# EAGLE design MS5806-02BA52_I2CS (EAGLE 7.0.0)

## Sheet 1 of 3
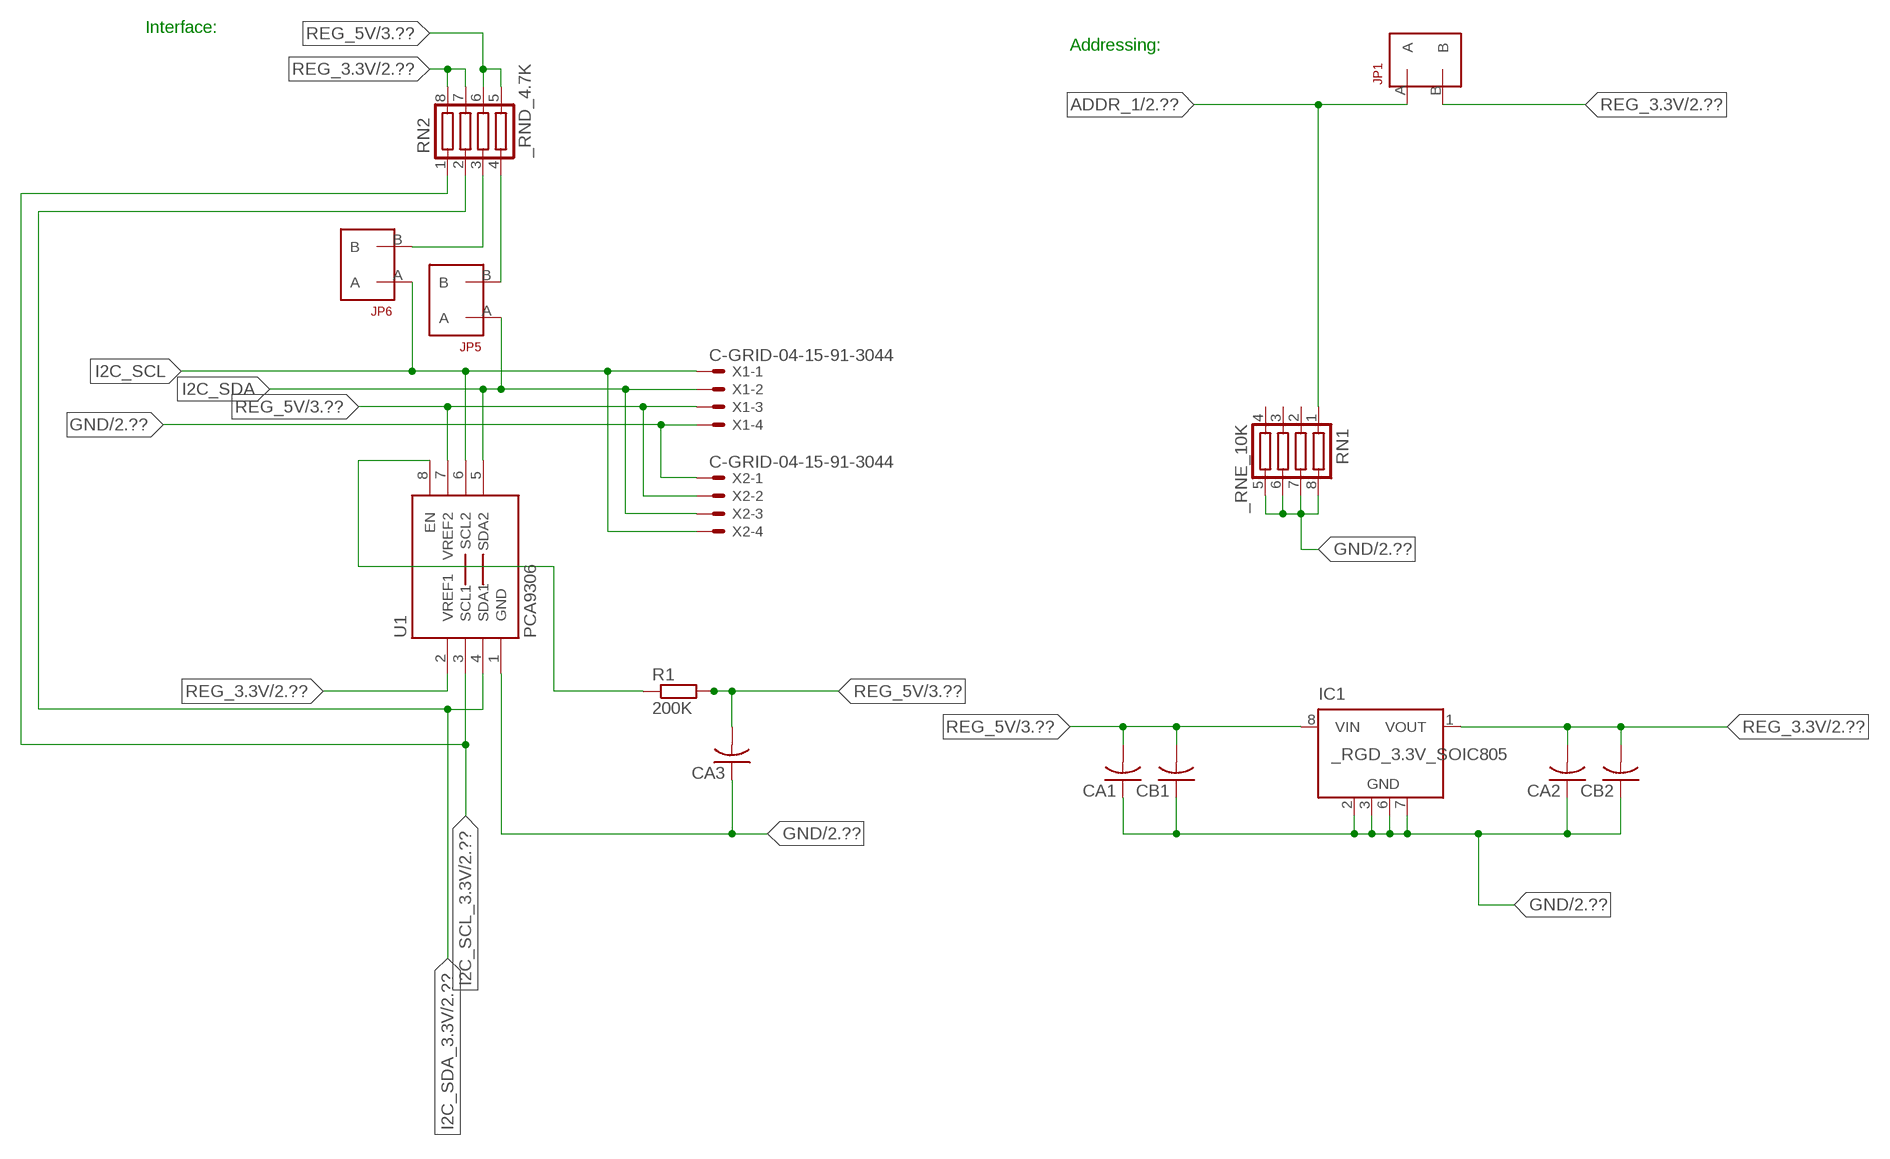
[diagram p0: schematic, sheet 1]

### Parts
CA1  CC1206KRX7R9BB104  [.1UF]
CA2  CC1206KRX7R9BB104  [.1UF]
CA3  CC1206KRX7R9BB104  [.1UF]
CB1  TMK316F106ZL-TC1206K  [TMK316F106ZL-T]
CB2  TMK316F106ZL-TC1206K  [TMK316F106ZL-T]
IC1  _RGD_3.3V_SOIC805  [_RGC_3.3V_SOIC8]
JP1  JUMPER_1X2_2MM  [JUMPER_1X2_2MM]
JP5  JUMPER_1X2_2MM  [JUMPER_1X2_2MM]
JP6  JUMPER_1X2_2MM  [JUMPER_1X2_2MM]
R1  200K  RESISTOR_SMT-0603  [R603]
RN1  _RNE_10K  [RNE]
RN2  _RND_4.7K  [RND]
U1  PCA9306  PCA9306_NCD  [PSOP-8]
X1  C-GRID-04-15-91-3044  [15-91-04]
X2  C-GRID-04-15-91-3044  [15-91-04]

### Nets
ADDR_1: JP1.A RN1.1 ; also sheet 2
GND: CA1.1 CA2.1 CA3.1 CB1.1 CB2.1 IC1.2(GND) IC1.3(GND) IC1.6(GND) IC1.7(GND) RN1.5 RN1.6 RN1.7 RN1.8 U1.1(GND) X1.4 X2.1 ; also sheet 2,3
I2C_SCL: JP6.A U1.6(SCL2) X1.1 X2.4
I2C_SCL_3.3V: RN2.1 U1.3(SCL1) ; also sheet 2
I2C_SDA: JP5.A U1.5(SDA2) X1.2 X2.3
I2C_SDA_3.3V: RN2.2 U1.4(SDA1) ; also sheet 2
N$1: JP6.B RN2.3
N$2: JP5.B RN2.4
N$3: R1.1 U1.8(EN)
REG_3.3V: CA2.2 CB2.2 IC1.1(VOUT) JP1.B RN2.7 RN2.8 U1.2(VREF1) ; also sheet 2
REG_5V: CA1.2 CA3.2 CB1.2 IC1.8(VIN) R1.2 RN2.5 RN2.6 U1.7(VREF2) X1.3 X2.2 ; also sheet 3
Unconnected: IC1.4(NC) IC1.5(NC) RN1.2 RN1.3 RN1.4

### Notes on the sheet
- Interface:
- Addressing:

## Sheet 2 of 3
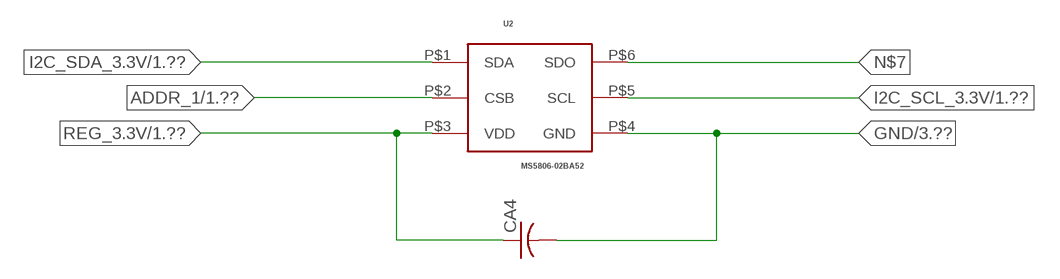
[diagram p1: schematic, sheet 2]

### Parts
CA4  _CA_.10UF_50VC1206K  [_CA_.1UF_50V]
U2  MS5806-02BA52  [MS5806-02BA52]

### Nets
ADDR_1: U2.P$2(CSB) ; also sheet 1
GND: CA4.2 U2.P$4(GND) ; also sheet 1,3
I2C_SCL_3.3V: U2.P$5(SCL) ; also sheet 1
I2C_SDA_3.3V: U2.P$1(SDA) ; also sheet 1
N$7: U2.P$6(SDO)
REG_3.3V: CA4.1 U2.P$3(VDD) ; also sheet 1

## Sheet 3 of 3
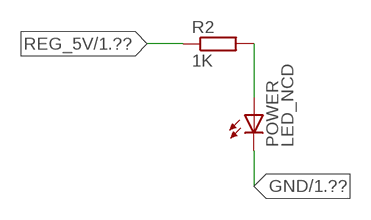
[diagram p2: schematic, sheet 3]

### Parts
POWER  LED_NCD  [CHIPLED_0603]
R2  1K  RESISTOR_SMT-0402  [R402]

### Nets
GND: POWER.C ; also sheet 1,2
N$4: POWER.A R2.2
REG_5V: R2.1 ; also sheet 1

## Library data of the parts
CA1-CA3 = NCD_ULTIMATE_LIBRARY:CC1206KRX7R9BB104: Capacitor CA .1uF 50V SMT C1206K CC1206KRX7R9BB104
CA4 = NCD_ULTIMATE_LIBRARY:_CA_.10UF_50V: Capacitor .1uF SMT
CB1 CB2 = NCD_ULTIMATE_LIBRARY:TMK316F106ZL-T: Capacitor CB 10uF SMT 1206 TMK316F106ZL-T
IC1 = NCD_ULTIMATE_LIBRARY:_RGD_3.3V_SOIC8: Regulator Linear 3.3V Chip Positive VOLTAGE REGULATOR Digikey 497-1199-2-ND/L78L33ACD13TR
JP1 JP5 JP6 = NCD_ULTIMATE_CONNECTORS:JUMPER_1X2_2MM
POWER = NCD_ULTIMATE_LIBRARY:LED_NCD: LED Digikey 754-1132-2-ND/APT2012SRCPRV
R1 R2 = NCD_ULTIMATE_LIBRARY:RESISTOR_SMT: NCD Resistor
RN1 = NCD_ULTIMATE_LIBRARY:_RNE_10K: Resistor Array RNE SMT 10K x 4 Single Resistor Source: http://www.ctscorp.com/components/Datasheets/CTSChipArrayDs.pdf Digikey 742C083103JPTR-ND/742C083103JP; OC_FARNELL: unknown; OC_NEWARK: unknown
RN2 = NCD_ULTIMATE_LIBRARY:_RND_4.7K: Resistor Array RND SMT 4.7K x 4 Single Resistor Source: http://www.ctscorp.com/components/Datasheets/CTSChipArrayDs.pdf Digikey 742C083472JPTR-ND/742C083472JP; OC_FARNELL: unknown; OC_NEWARK: unknown
U1 = NCD_ULTIMATE_LIBRARY:PCA9306_NCD: NCD Bidirectional I2C level shifter. NOT compatible with all available part number pinout schemes- DOUBLE CHECK!!!; PROD_ID: IC-10023
U2 = NCD_ULTIMATE_bhaskar:MS5806-02BA52
X1 X2 = NCD_ULTIMATE_CONNECTORS:C-GRID-04: CONNECTOR 4-Pos I2C wire to board 2.54 mm (0.100") pitch header Digikey WM1342-ND/0015912045; OC_FARNELL: unknown; OC_NEWARK: unknown

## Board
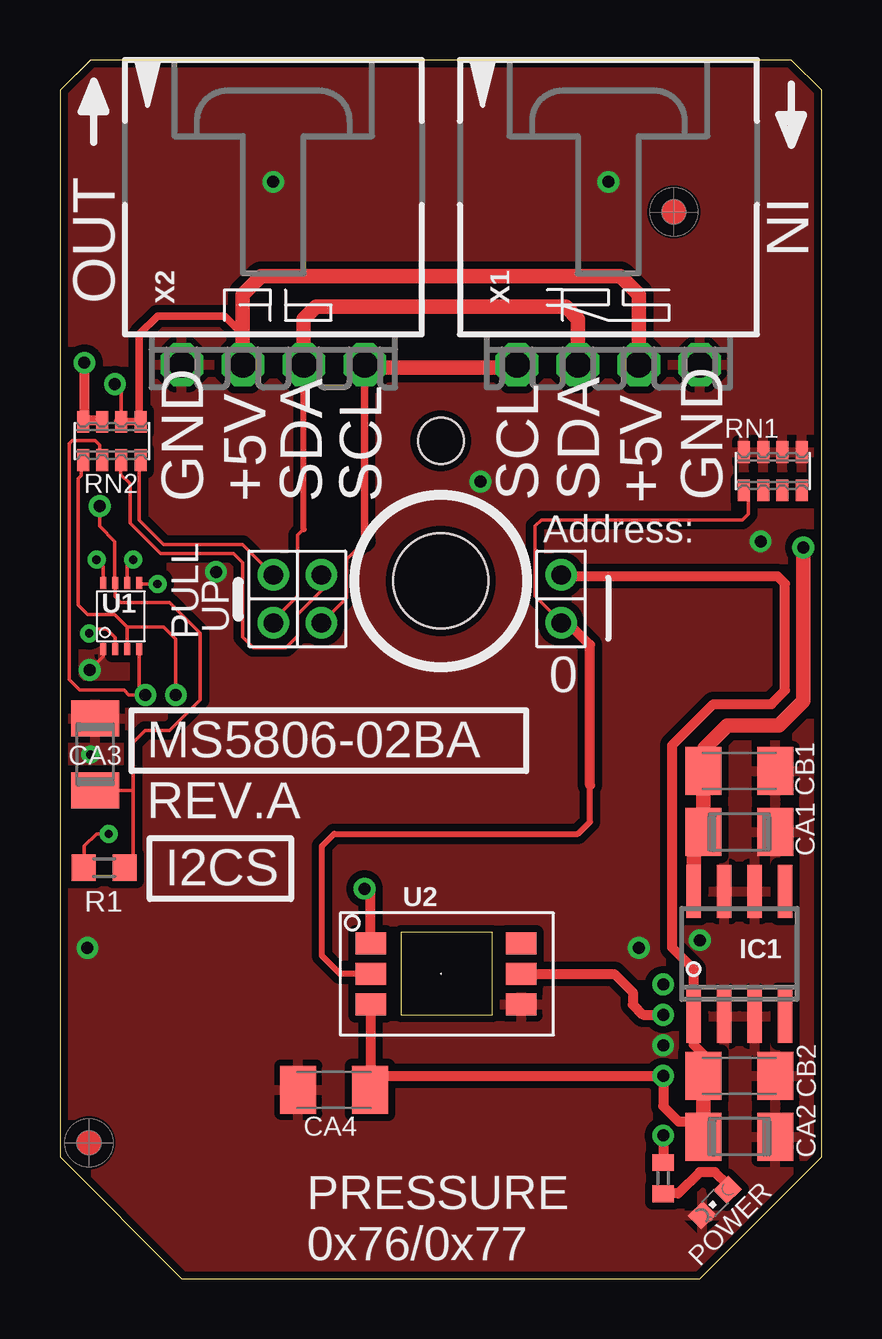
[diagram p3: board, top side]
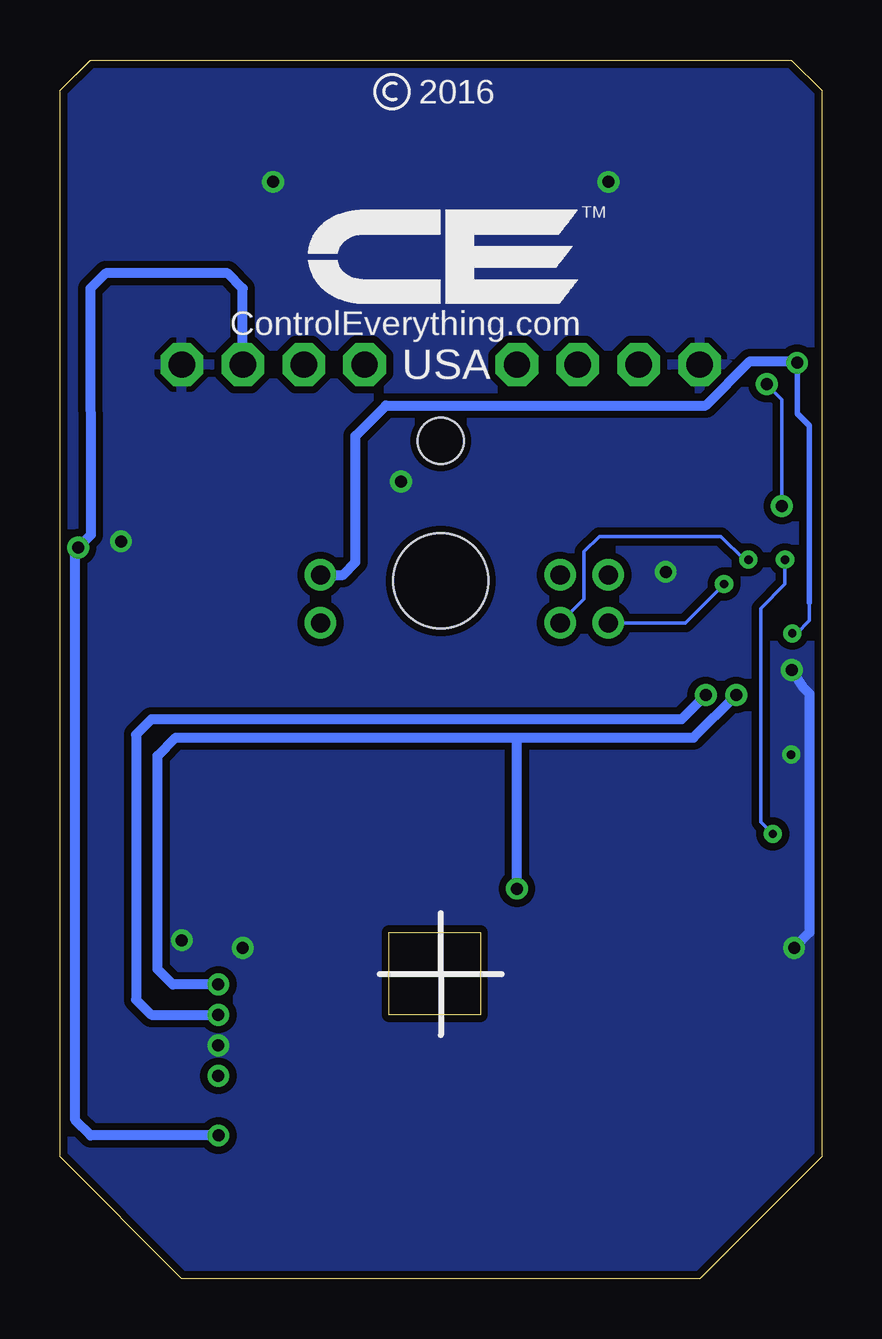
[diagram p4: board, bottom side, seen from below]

Size 31.75 x 50.8 mm. Coordinates in mm from the lower left corner, seen from the top.
Outline: 32 segments
Copper layers (1*16): Top 0.035mm / dielectric 1.5mm / Bottom 0.035mm
Design rules "default": minimum track width 5mil, minimum drill 24mil, track to track 5mil, track to pad 5mil, pad to pad 5mil, via to via 5mil, smd to smd 5mil, copper to edge 10mil, drill to drill 8mil, minimum pad ring 10mil, minimum via ring 8mil, stop-mask expansion 2mil, vias tented up to drill 0mil, thermal gap 10mil
Holes 3.96 mm at 15.88,29.08
Holes 1.91 mm at 15.88,34.93

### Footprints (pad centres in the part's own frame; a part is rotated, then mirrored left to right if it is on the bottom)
.1UF = smd 1.5 x 2: 1 -1.5,0; 2 1.5,0
_CA_.1UF_50V = smd 1.5 x 2: 1 -1.5,0; 2 1.5,0
TMK316F106ZL-T = smd 1.5 x 2: 1 -1.5,0; 2 1.5,0
_RGC_3.3V_SOIC8 = smd 0.6 x 2.2: 1 -1.905,-2.6; 2 -0.635,-2.6; 3 0.635,-2.6; 4 1.905,-2.6; 5 1.905,2.6; 6 0.635,2.6; 7 -0.635,2.6; 8 -1.905,2.6
JUMPER_1X2_2MM = drill 0.8: A 0,2; B 0,0
CHIPLED_0603 = smd 0.8 x 0.876: A 0,-0.75; C 0,0.75
R603 = smd 1 x 1.1: 1 -0.85,0; 2 0.85,0
R402 = smd 0.7 x 0.9: 1 -0.65,0; 2 0.65,0
RNE = smd 0.5 x 0.9: 1 -1.2,-0.8; 2 -0.4,-0.8; 3 0.4,-0.8; 4 1.2,-0.8; 5 1.2,0.8; 6 0.4,0.8; 7 -0.4,0.8; 8 -1.2,0.8
RND = smd 0.5 x 0.9: 1 -1.2,-0.8; 2 -0.4,-0.8; 3 0.4,-0.8; 4 1.2,-0.8; 5 1.2,0.8; 6 0.4,0.8; 7 -0.4,0.8; 8 -1.2,0.8
PSOP-8 = smd 0.25 x 0.5: 1 -0.73,-1.37; 2 -0.23,-1.37; 3 0.27,-1.37; 4 0.77,-1.37; 5 0.77,1.38; 6 0.27,1.38; 7 -0.23,1.38; 8 -0.73,1.38
MS5806-02BA52 = smd 1.27 x 0.92: P$1 -2.54,2.54; P$2 -2.54,1.27; P$3 -2.54,0; P$4 3.74,0; P$5 3.74,1.27; P$6 3.74,2.54
15-91-04 = drill 1.1 pad 1.778 octagon: 1 -3.81,-7.62; 2 -1.27,-7.62; 3 1.27,-7.62; 4 3.81,-7.62

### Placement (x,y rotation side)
CA1  28.32,18.62 180 top
CA2  28.32,5.92 180 top
CA3  1.46,21.86 270 top
CA4  11.43,7.87 180 top
CB1  28.32,21.16 180 top
CB2  28.32,8.46 180 top
IC1  28.32,13.54 0 top
JP1  20.89,29.34 180 top
JP5  8.89,29.34 180 top
JP6  10.9,29.34 180 top
POWER  27.3,3.18 135 top
R1  1.84,17.13 0 top
R2  25.15,4.19 270 top
RN1  29.72,33.66 0 top
RN2  2.16,34.93 0 top
U1  2.54,27.61 0 top
U2  15.49,11.43 0 top
U$5  [VISION_REF10]  1.21,5.66 90 top
U$28  [VISION_REF10]  25.59,44.46 90 top
X1  22.86,45.72 0 top
X2  8.89,45.72 0 top

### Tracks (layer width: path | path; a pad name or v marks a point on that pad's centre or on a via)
ADDR_1
  Top 0.152: JP1.A 20.89,27.37 19.81,28.45 19.81,31.37 20.07,31.62 28.45,31.62 28.7,31.88 28.7,32.78 RN1.1
  Top 0.254: U2.P$2 11.68,12.7 10.92,13.46 10.92,18.03 11.43,18.54 21.59,18.54 22.1,19.05 22.1,20.57
  Top 0.406: 22.1,20.57 22.1,26.42 21.18,27.34 JP1.A
GND  (via drill 0.35, 0.5)
  Top 0.152: CA3.1 1.52,23.42 1.52,23.62 | v1.25,25.38 1.81,25.94 U1.1
  Bottom 0.406: v1.25,25.38 0.76,24.64 0.51,24.38 0.51,14.43 v1.15,13.79
  other vias: 8.89,45.72 22.86,45.72 25.15,9.73 17.53,33.22 26.67,14.11 6.5,29.46 29.21,30.73 1.27,21.84 24.13,13.79
  pour Bottom (isolate 0.305): -0.64,5.08 -0.64,49.53 1.27,51.44 30.48,51.44 32.38,49.53 32.38,5.08 26.67,-0.63 5.08,-0.63
  pour Top (isolate 0.305): 4.45,-1.27 -1.27,4.45 -1.27,50.17 0.64,52.07 31.11,52.07 33.02,50.17 33.02,4.45 27.3,-1.27
I2C_SCL  (via drill 0.35)
  Top 0.152: 12.7,30.73 11.94,29.97 11.94,28.38 JP6.A | v3.05,29.97 2.81,29.73 U1.6
  Top 0.305: 12.7,30.73 X2.4
  Top 0.406: X2.4 12.7,37.97 | 19.05,37.97 X1.1
  Top 0.61: 12.7,37.97 19.05,37.97
  Bottom 0.152: JP6.A 9.91,28.33 9.91,30.3 9.27,30.94 4.19,30.94 3.23,29.97 v3.05,29.97
I2C_SCL_3.3V  (via drill 0.5)
  Top 0.152: RN2.1 0.89,34.07 0.89,33.48 0.77,33.35 0.77,28.08 1.16,27.69 2.29,27.69 2.81,27.17 | 2.81,27.17 U1.3 | v4.83,24.33 v4.83,24.34 4.83,26.67 4.33,27.17 2.81,27.17
  Top 0.406: U2.P$5 23.11,12.7 23.88,11.94 23.88,11.43 24.31,11 v25.15,11
  Bottom 0.406: v4.83,24.33 5.84,23.32 27.94,23.32 28.58,22.68 28.58,11.63 27.94,11 v25.15,11
I2C_SDA  (via drill 0.35)
  Top 0.152: JP5.A 8.89,27.44 9.91,28.45 9.91,30.99 10.16,31.24 | U1.5 3.34,28.96 v4.06,28.96
  Top 0.254: 10.16,31.24 10.16,31.25 X2.3
  Top 0.61: X2.3 10.16,40.01 10.67,40.51 21.09,40.51 21.59,40.01 X1.2
  Bottom 0.152: v4.06,28.96 5.68,27.34 JP5.A
I2C_SDA_3.3V  (via drill 0.5)
  Top 0.152: RN2.2 1.65,34.14 1.65,34.75 1.46,34.94 0.51,34.94 0.38,34.81 0.38,26.37 0.38,26.36 0.38,24.97 0.81,24.54 2.67,24.54 2.87,24.33 v3.56,24.33 3.31,24.58 U1.4
  Top 0.406: U2.P$1 12.95,16.26 v12.7,16.26
  Bottom 0.406: v25.15,12.27 27.05,12.27 27.69,12.9 27.69,21.79 26.93,22.56 12.7,22.56 | 12.7,22.56 5.34,22.56 v3.56,24.33 | v12.7,16.26 12.7,22.56
N$1
  Top 0.152: JP6.B 10.92,29.31 10.92,28.7 9.91,27.69 9.91,26.8 9.42,26.31 8.06,26.31 7.62,26.75 7.62,29.84 7.24,30.23 4.19,30.23 2.92,31.5 2.92,33.15 2.54,33.53 2.54,34.1 RN2.3
  Top 0.305: 2.54,34.02 RN2.3
N$2
  Top 0.152: JP5.B 7.62,30.61 4.32,30.61 3.3,31.62 3.3,34.07 RN2.4
  Top 0.305: 3.37,33.88 RN2.4
N$3  (via drill 0.35)
  Top 0.152: R1.1 1.02,17.16 1.02,18.03 1.52,18.54 v2.03,18.54 | v1.52,29.97 1.81,29.69 U1.8
  Bottom 0.152: v2.03,18.54 2.54,19.05 2.54,27.94 1.52,28.96 v1.52,29.97
N$4
  Top 0.406: POWER.A 27.84,3.92 27.3,4.45 26.67,4.45 25.78,3.56 25.16,3.56 R2.2
REG_3.3V  (via drill 0.35, 0.5)
  Top 0.152: v1.22,26.9 1.4,27.08 1.96,27.08 2.31,26.73 U1.2
  Top 0.406: CB2.2 26.82,9.35 26.42,9.75 26.42,10.36 | 26.82,6.55 25.78,6.55 25.15,7.19 v25.15,8.46 13.11,8.46 CA4.1 12.95,9.12 U2.P$3 | IC1.1 26.42,12.9 25.53,13.79 25.53,22.24 27.24,23.95 29.66,23.95 30.23,24.52 30.23,28.97 29.91,29.29 20.95,29.29 JP1.B | 26.52,5.62 CA2.2 | v1.02,38.18 1.02,35.78 | 1.02,35.78 RN2.8 | 1.02,35.78 1.71,35.78 RN2.7
  Top 0.61: CB2.2 26.82,6.55 CA2.2 | 26.42,10.36 IC1.1
  Bottom 0.152: 0.51,28.19 0.51,27.43 1.04,26.9 v1.22,26.9
  Bottom 0.229: 0.51,28.19 0.51,35.56 1.02,36.07 v1.02,38.18
  Bottom 0.406: v1.02,38.18 1.08,38.24 2.99,38.24 4.83,36.4 18.16,36.4 19.43,35.13 19.43,29.87 19.94,29.34 JP1.B
REG_5V  (via drill 0.5)
  Top 0.152: RN2.6 2.56,37.01 v2.29,37.29 | R1.2 3.05,17.49 3.05,20.36 | 3.05,20.36 3.05,22.35 3.56,22.86 4.57,22.86 5.84,24.13 5.84,26.92 4.57,28.19 2.54,28.19 2.31,28.43 U1.7 2.29,29.01 2.29,30.73 1.65,31.37 v1.65,32.21 | CA3.2 3.05,20.36
  Top 0.305: 7.62,39.37 7.5,39.37 | 2.42,35.74 RN2.6 RN2.5 3.31,35.8 3.31,39.37 4.07,40.13 6.86,40.13 7.62,39.37 | X2.2 7.62,39.37
  Top 0.406: v25.15,5.97 R2.1
  Top 0.61: X1.3 24.13,41.02 23.37,41.78 8.38,41.78 7.62,41.02 X2.2 | IC1.8 26.42,18.21 CA1.2 CB1.2 26.86,21.2 26.86,22.11 27.82,23.06 29.98,23.06 30.99,24.08 v30.99,30.48
  Bottom 0.152: v1.65,32.21 1.65,36.65 v2.29,37.29
  Bottom 0.406: X1.3 24.13,41.28 24.77,41.91 29.84,41.91 30.48,41.27 30.47,31 v30.99,30.48 31.11,30.36 31.11,6.6 30.48,5.97 v25.15,5.97

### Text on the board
tNames: IN | OUT | GND | +5V | SDA | SCL | SCL | SDA | +5V | GND | Address: | PULL | UP | 0 | MS5806-02BA | REV.A | I2CS | PRESSURE / 0x76/0x77
bNames: 2016 | TM | ControlEverything.com | USA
